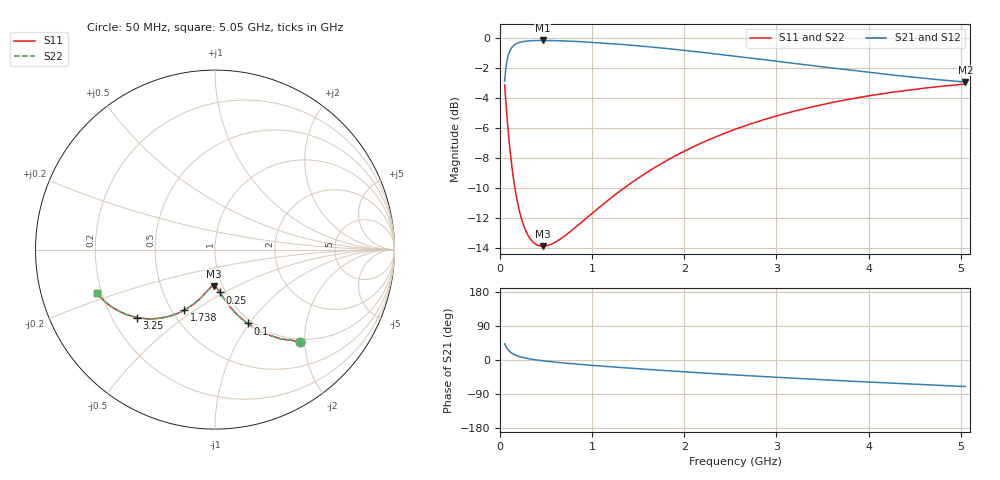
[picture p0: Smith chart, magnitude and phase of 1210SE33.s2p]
! AVX Thin Film Operation		Date: August 2001
! Description: Accu-P® Series, Thin Film, SMD, RF Capacitor
! Part Number: 12101J330FBT
! 50 MHz  -  5.05 GHz
! Serial Measurements
# mhz S db R 50
!	S11		S21		S12		S22
!	dB	Phase	dB	Phase	dB	Phase	dB	Phase
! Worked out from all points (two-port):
!   401 points, 50 MHz to 5.05 GHz, reference 50 ohm
!   highest |S21| = -0.18 dB at 462.5 MHz (marker M1); lowest = -3.0 dB at 5.05 GHz (marker M2)
!   |S21| within 3 dB of the highest: start of sweep to end of sweep
!   lowest |S11| = -13.9 dB at 462.5 MHz (marker M3), VSWR 1.51, Z = 45.5 - j19.2 ohm
!   |S11| at or under -10 dB: 161.6 MHz to 1.347 GHz (1.185 GHz wide, 157 % of centre)
!   |S22| runs from -13.9 to -3.1 dB; largest |S21 - S12| = 0
!   S11 on the Smith chart (normalised r, x): 50 MHz: 0.95, -1.90; 100 MHz: 0.95, -0.98; 250 MHz: 0.94, -0.48; 1.738 GHz: 0.58, -0.45; 3.25 GHz: 0.30, -0.34; 5.05 GHz: 0.18, -0.17
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50  -3.14 -47.3  -2.89 42.7  -2.89 42.7  -3.14 -47.3
75  -5.20 -58.9  -1.56 31.1  -1.56 31.1  -5.20 -58.9
87.5  -6.11 -62.9  -1.22 27.1  -1.22 27.1  -6.11 -62.9
100  -6.95 -66.2  -0.98 23.7  -0.98 23.7  -6.95 -66.2
125  -8.38 -71.3  -0.68 18.7  -0.68 18.7  -8.38 -71.3
150  -9.54 -74.9  -0.51 15.0  -0.51 15.0  -9.54 -74.9
200  -11.25 -80.0  -0.34 10.0  -0.34 10.0  -11.25 -80.0
250  -12.38 -83.4  -0.26 6.5  -0.26 6.5  -12.38 -83.5
300  -13.10 -86.1  -0.22 3.9  -0.22 3.9  -13.10 -86.1
350  -13.54 -88.2  -0.20 1.8  -0.20 1.8  -13.54 -88.2
462.5  -13.87 -91.9  -0.18 -2.0  -0.18 -2.0  -13.87 -91.9
625  -13.52 -96.2  -0.20 -6.3  -0.20 -6.3  -13.52 -96.2
887.5  -12.27 -101.9  -0.27 -11.9  -0.27 -11.9  -12.27 -101.9
1287.5  -10.27 -109.4  -0.43 -19.4  -0.43 -19.4  -10.27 -109.4
1725  -8.47 -116.8  -0.67 -26.8  -0.67 -26.8  -8.47 -116.8
1737.5  -8.43 -117.0  -0.68 -27.0  -0.68 -27.0  -8.43 -117.0
2137.5  -7.14 -123.3  -0.94 -33.3  -0.94 -33.3  -7.14 -123.3
2550  -6.10 -129.4  -1.23 -39.4  -1.23 -39.4  -6.10 -129.4
3250  -4.80 -138.9  -1.75 -48.9  -1.75 -48.9  -4.80 -138.9
3387.5  -4.60 -140.6  -1.86 -50.7  -1.86 -50.7  -4.60 -140.6
4225  -3.66 -150.7  -2.46 -60.8  -2.46 -60.8  -3.66 -150.7
5050  -3.08 -159.9  -2.95 -69.9  -2.95 -69.9  -3.08 -159.9
